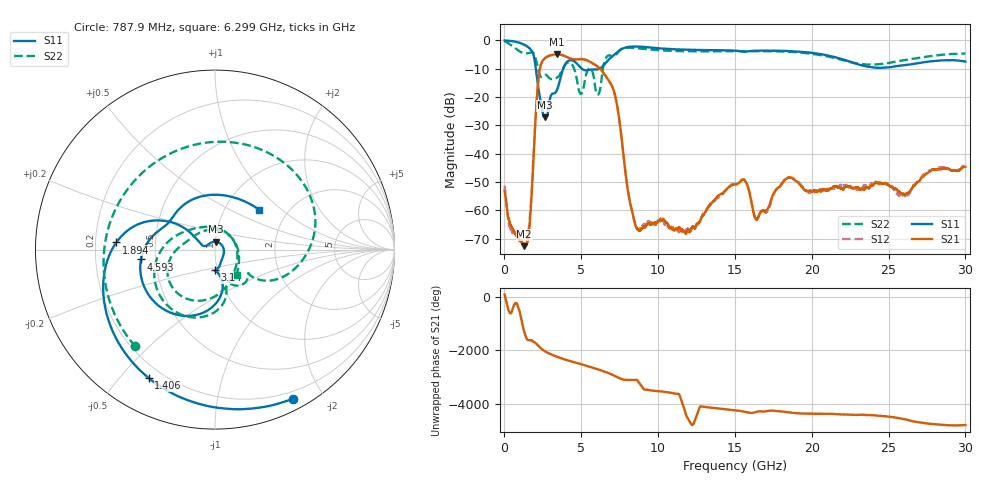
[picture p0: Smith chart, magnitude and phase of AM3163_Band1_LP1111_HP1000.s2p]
!Agilent Technologies,E8364B,MY43040894,A.07.50.67
!Agilent E8364B: A.07.50.67
!Date: Thursday, August 20, 2020 12:00:50
!Correction: S11(Full 2 Port(1,2))
!S21(Full 2 Port(1,2))
!S12(Full 2 Port(1,2))
!S22(Full 2 Port(1,2))
!S2P File: Measurements: S11, S21, S12, S22:
# Hz S  dB  R 50
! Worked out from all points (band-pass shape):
!   3201 points, 10 MHz to 30 GHz, reference 50 ohm
!   highest |S21| = -4.92 dB at 3.44 GHz (marker M1); lowest = -72.6 dB at 1.285 GHz (marker M2)
!   |S21| within 3 dB of the highest: 2.411 GHz to 5.686 GHz (3.275 GHz wide, 80.9 % of centre)
!   lowest |S11| = -27.2 dB at 2.634 GHz (marker M3), VSWR 1.09, Z = 50.2 + j4.39 ohm
!   |S11| at or under -10 dB: 2.042 GHz to 3.824 GHz (1.781 GHz wide, 60.7 % of centre); 5.042 GHz to 6.18 GHz (1.137 GHz wide, 20.3 % of centre)
!   |S22| runs from -19.2 to -0.3 dB; largest |S21 - S12| = 0.0048
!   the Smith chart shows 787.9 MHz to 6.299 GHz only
!   S11 on the Smith chart (normalised r, x): 787.9 MHz: 0.12, -1.65; 1.406 GHz: 0.15, -0.60; 1.894 GHz: 0.29, +0.03; 3.14 GHz: 0.97, -0.23; 4.593 GHz: 0.41, -0.06; 6.299 GHz: 1.44, +0.72
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1e7  -0.02 -5.5  -52.99 95.6  -51.26 -115.8  -0.29 -12.2
7.878656e8  -0.56 -62.4  -69.05 135.4  -68.75 -63.3  -3.11 -129.4
1.284575e9  -1.53 -105.5  -72.61 134.7  -71.92 107.9  -4.54 148.0
1.406409e9  -1.88 -117.3  -72.27 -70.1  -71.77 11.1  -4.60 126.1
1.893747e9  -5.17 175.9  -41.08 124.4  -40.70 126.2  -4.49 22.2
2.231134e9  -17.67 148.4  -12.79 -42.8  -12.79 -42.8  -11.05 -35.3
2.634125e9  -27.16 85.3  -6.28 125.9  -6.29 125.9  -12.14 -44.9
3.140206e9  -18.78 -90.4  -5.07 -18.3  -5.08 -18.4  -13.59 -67.9
3.440106e9  -17.23 -81.1  -4.92 -86.2  -4.93 -86.2  -13.08 -73.5
3.9087e9  -8.91 -100.8  -5.49 179.7  -5.50 179.8  -8.92 -92.9
4.592847e9  -7.61 -172.4  -6.72 66.7  -6.70 66.8  -10.93 176.0
5.014581e9  -9.87 158.9  -6.60 -2.3  -6.58 -2.5  -18.78 25.5
6.298528e9  -9.59 42.2  -10.43 123.1  -10.49 123.0  -14.57 -49.6
7.498128e9  -3.49 -100.9  -28.94 -170.3  -28.90 -169.2  -3.46 -168.9
8.547778e9  -2.15 177.0  -65.56 132.5  -65.43 132.0  -2.73 127.9
1.000979e10  -2.76 100.7  -63.82 64.3  -63.61 71.6  -3.45 65.7
1.227778e10  -3.36 9.8  -65.66 -106.1  -65.88 -108.8  -3.84 -14.9
1.5005e10  -3.59 -73.9  -50.88 67.2  -50.56 67.3  -3.79 -92.4
2.000958e10  -4.39 162.8  -53.21 -56.7  -53.65 -43.4  -4.70 135.7
2.274617e10  -7.98 59.9  -52.18 -103.1  -52.51 -95.2  -7.94 20.5
2.500479e10  -9.51 -62.9  -51.01 -170.8  -50.47 -173.3  -7.97 -93.2
3e10  -7.48 105.5  -44.62 -124.6  -43.91 -130.6  -4.62 101.1
